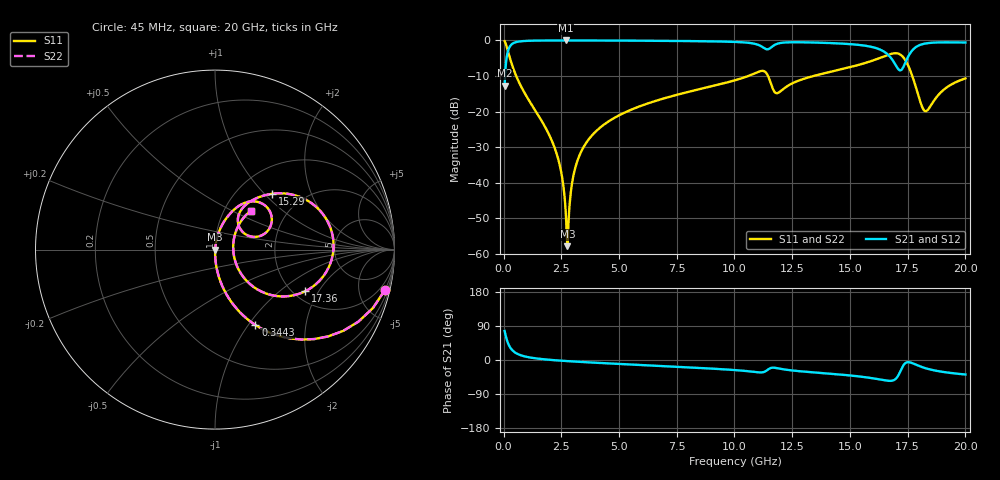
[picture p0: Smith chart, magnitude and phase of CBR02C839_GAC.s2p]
! S-parameter model data by Modelithics Inc.  support@modelithics.com 813-866-6335  Tampa FL USA
! S-Parameter data specifications:
! Substrate: 20-mil Rogers 4350B, substrate thickness, H=0.508mm, Dielectric constant, Er=3.75
! PCB Mounting Pad Footprint: Pad width, PadW=0.32mm , Pad length, PadL=0.37mm , Pad gap, PadG (edge-to-edge)=0.19mm , Reference planes=0.93mm apart
#  GHz  S  MA  R 50
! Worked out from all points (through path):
!   801 points, 45 MHz to 20 GHz, reference 50 ohm
!   highest |S21| = -0.01 dB at 2.689 GHz (marker M1); lowest = -12.7 dB at 45 MHz (marker M2)
!   group delay of S21, straight-line fit = 6.87 ps
!   lowest |S11| = -57.8 dB at 2.764 GHz (marker M3), VSWR 1.00, Z = 50.1 - j0.00472 ohm
!   |S11| at or under -10 dB: 547.5 MHz to 10.59 GHz (10.05 GHz wide, 180 % of centre); 11.45 GHz to 13.42 GHz (1.966 GHz wide, 15.8 % of centre); 17.7 GHz to end of sweep
!   |S22| runs from -57.8 to -0.2 dB; largest |S21 - S12| = 0
!   S11 on the Smith chart (normalised r, x): 45 MHz: 0.99, -8.41; 344.3 MHz: 0.99, -1.08; 15.29 GHz: 1.43, +1.11; 17.36 GHz: 2.31, -1.54; 20 GHz: 1.33, +0.63
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0.045  0.973 -13.4  0.2305 76.6  0.2305 76.6  0.973 -13.4
0.194662  0.6965 -46.0  0.7171 43.9  0.7171 43.9  0.6965 -46.0
0.344325  0.4772 -61.8  0.8782 28.1  0.8782 28.1  0.4772 -61.8
0.818256  0.2073 -78.7  0.9774 11.1  0.9774 11.1  0.2073 -78.7
2.215106  0.03082 -88.4  0.9983 -0.6  0.9983 -0.6  0.03082 -88.4
2.514431  0.01315 -86.5  0.9986 -1.9  0.9986 -1.9  0.01315 -86.5
2.689037  0.003995 -74.0  0.9987 -2.6  0.9987 -2.6  0.003995 -74.0
2.763869  0.001291 -2.1  0.9987 -2.9  0.9987 -2.9  0.001291 -2.1
3.03825  0.01325 80.2  0.9985 -4.0  0.9985 -4.0  0.01325 80.2
3.387462  0.02857 82.0  0.9981 -5.2  0.9981 -5.2  0.02857 82.0
4.534875  0.07249 79.8  0.9957 -9.0  0.9957 -9.0  0.07249 79.8
6.704981  0.1454 73.7  0.9872 -15.5  0.9872 -15.5  0.1454 73.7
10.0225  0.2756 61.5  0.9522 -26.6  0.9522 -26.6  0.2756 61.5
11.24474  0.3729 35.3  0.7953 -32.1  0.7953 -32.1  0.3729 35.3
11.84339  0.1816 37.9  0.8951 -21.5  0.8951 -21.5  0.1816 37.9
13.36496  0.3129 55.0  0.9353 -32.4  0.9353 -32.4  0.3129 55.0
15.28563  0.4449 44.3  0.8717 -42.6  0.8717 -42.6  0.4449 44.3
16.68248  0.632 18.4  0.6147 -55.0  0.6147 -55.0  0.632 18.4
17.35596  0.5542 -24.7  0.4528 -10.8  0.4528 -10.8  0.5542 -24.7
17.78001  0.2646 -44.6  0.77 -10.3  0.77 -10.3  0.2646 -44.6
18.25394  0.1018 -1.8  0.9031 -21.3  0.9031 -21.3  0.1018 -1.8
20  0.293 47.4  0.9336 -38.3  0.9336 -38.3  0.293 47.4
